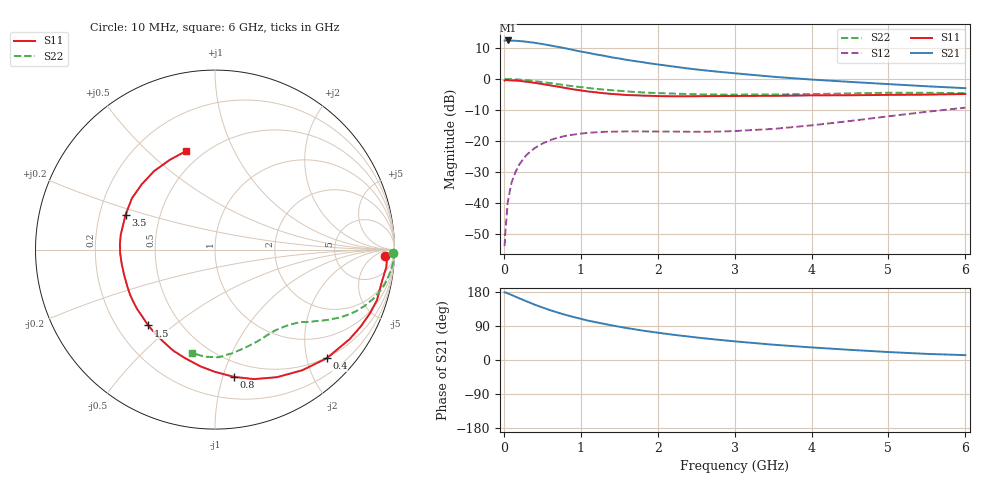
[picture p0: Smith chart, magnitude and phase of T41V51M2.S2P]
! Infineon Technologies  Discrete & RF Semiconductors
! BFR182T
! Si NPN RF Bipolar Junction Transistor in SC75
! VCE = 1.5 V  IC = 1.2 mA
! Common Emitter S-Parameters:  October  1999
# GHz  S  MA  R  50
!  f  S11  S21  S12  S22
! GHz  MAG  ANG  MAG  ANG  MAG  ANG  MAG  ANG
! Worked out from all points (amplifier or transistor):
!   36 points, 10 MHz to 6 GHz, reference 50 ohm
!   highest |S21| = 12.4 dB at 50 MHz (marker M1)
!   |S21| within 3 dB of that: start of sweep to 889.1 MHz
!   unconditionally stable (mu >= 1): 2.249 GHz to 4.622 GHz
!   at 250 MHz: K = 0.12, MSG = 19.0 dB, |S12| = -25.9 dB
!   at 1.4 GHz: K = 0.64, MSG = 12.0 dB, |S12| = -17.0 dB
!   at 6 GHz: K = 0.86, MSG = 3.1 dB, |S12| = -9.2 dB
!   S11 on the Smith chart (normalised r, x): 10 MHz: 24, -17; 400 MHz: 0.48, -2.38; 800 MHz: 0.37, -1.09; 1.5 GHz: 0.33, -0.41; 3.5 GHz: 0.31, +0.17; 6 GHz: 0.41, +0.67
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0.01  0.946 -2.2  4.159 178.6  0.002 84.3  0.9912 -1.2
0.02  0.9604 -1.1  4.174 178.6  0.0034 100.9  0.9944 -0.9
0.05  0.9595 -5.8  4.191 175.7  0.0102 86.0  0.9961 -2.4
0.1  0.9464 -11.1  4.156 171.8  0.0213 83.8  0.9941 -4.6
0.2  0.9332 -22.5  4.102 162.8  0.0416 77.7  0.9767 -9.1
0.3  0.9012 -33.5  3.984 154.4  0.0604 71.0  0.9545 -13.3
0.4  0.8685 -44.2  3.844 146.1  0.0765 64.6  0.9244 -17.2
0.5  0.8297 -54.1  3.671 138.7  0.0904 59.6  0.8918 -20.5
0.6  0.7903 -64.1  3.485 131.6  0.103 54.8  0.8593 -23.5
0.7  0.7537 -73.2  3.307 125.2  0.1129 50.7  0.8251 -26.1
0.8  0.7166 -81.6  3.135 119.2  0.1205 47.0  0.7942 -28.4
0.9  0.6805 -90.2  2.947 113.7  0.1263 43.8  0.7637 -30.3
1.1  0.6273 -105.4  2.641 103.6  0.1355 38.7  0.7156 -33.6
1.3  0.589 -119.1  2.376 95.4  0.1404 35.2  0.6744 -36.4
1.5  0.563 -131.4  2.142 87.8  0.1417 33.0  0.6449 -38.7
1.8  0.5397 -147.9  1.872 77.7  0.1425 30.9  0.6076 -42.4
2.2  0.5256 -164.4  1.592 66.7  0.1416 31.5  0.5812 -47.0
2.8  0.5306 176.4  1.306 53.2  0.1417 36.9  0.5594 -55.2
3.5  0.5349 158.7  1.087 40.4  0.1562 46.7  0.5633 -65.0
4.5  0.5468 138.2  0.898 26.8  0.2099 56.1  0.5847 -80.2
5.5  0.56 116.7  0.763 16.1  0.2958 56.6  0.5996 -95.4
6  0.5721 106.4  0.711 12.8  0.3448 53.9  0.59 -102.6
